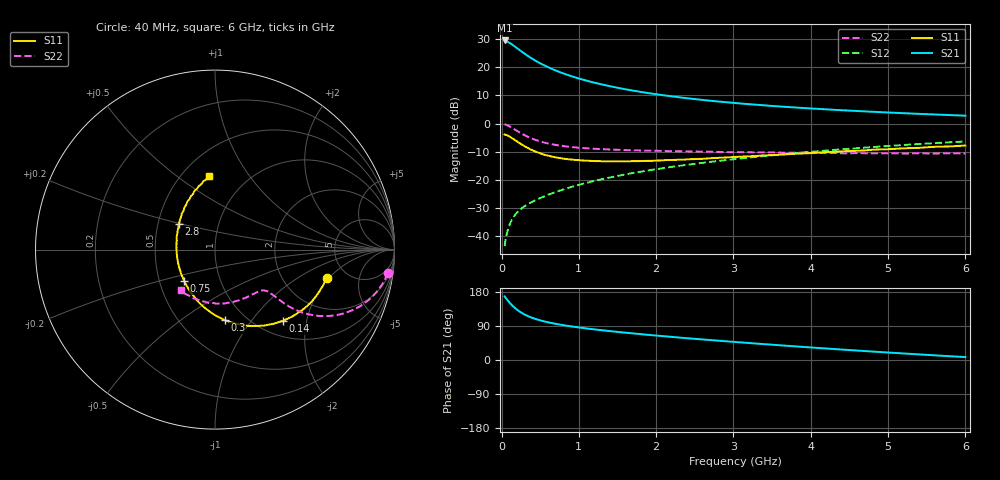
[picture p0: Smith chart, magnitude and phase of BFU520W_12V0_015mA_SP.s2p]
! Filename:  P:\Prog\Test\Noise\ATS_data\Testdata_Net\Run2\BFU520W_APM2013_06_A05_12p0V_015mA_SP_CM01_D.s2p
! Date/Time: Tue 26/Mar/2013 18:01:44
! BFU520W_APM2013_06_A05_12p0V_1to20mA_SP_CM01_Bias7_R.s2p
! MDIF S-parameter v. bias file
! BFU520W_APM2013_06_A05_12p0V_1to20mA_SP_CM01
! Date/time Thu Mar 21 16:35:01 2013
! VAR V_out= 12.0000
! VAR I_out= 14.9950
! VAR V_in= 0.7974
! VAR I_in= 0.1535
! Device data file deembeded for feedlines and parallel
! Original file: \Run2\BFU520W_APM2013_06_A05_12p0V_015mA_SP_CM01_R.s2p
! Feed-files: PR019V01_070313_Feed1.s2p, PR019V01_070313_Feed2.s2p
! Parallel-file: PR019V01_070313_Par.s2p
# MHz S MA R 50
!  Freq-MHz  S11-mag  S11-arg  S21-mag  S21-arg  S12-mag  S12-arg  S22-mag  S22-arg
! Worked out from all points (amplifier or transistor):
!   98 points, 40 MHz to 6 GHz, reference 50 ohm
!   highest |S21| = 29.4 dB at 40 MHz (marker M1)
!   |S21| within 3 dB of that: start of sweep to 214.3 MHz
!   unconditionally stable (mu >= 1): 1.331 GHz to 2.538 GHz
!   at 300 MHz: K = 0.60, MSG = 27.0 dB, |S12| = -29.3 dB
!   at 1.6 GHz: K = 1.01, MAG = 14.5 dB, |S12| = -18.0 dB
!   at 6 GHz: K = 0.88, MSG = 4.6 dB, |S12| = -6.3 dB
!   S11 on the Smith chart (normalised r, x): 40 MHz: 3.50, -1.87; 140 MHz: 1.28, -1.46; 300 MHz: 0.80, -0.75; 750 MHz: 0.67, -0.25; 2.8 GHz: 0.64, +0.20; 6 GHz: 0.68, +0.66
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40  0.6411 -14.2  29.66 167.8  0.006734 82.5  0.97 -7.7
50  0.6355 -17.8  29.56 165.0  0.008316 81.4  0.9625 -9.8
90  0.602 -31.4  27.52 154.8  0.0142 76.3  0.9125 -16.9
120  0.5699 -40.8  26.09 147.8  0.0181 73.2  0.8672 -21.4
140  0.5482 -46.5  24.95 143.6  0.02044 71.5  0.8347 -24.0
180  0.5039 -57.1  22.74 136.2  0.02466 68.7  0.7722 -28.1
220  0.4636 -66.4  20.73 129.8  0.02822 67.1  0.7149 -31.2
260  0.4267 -74.6  18.88 124.4  0.03144 66.0  0.664 -33.5
300  0.3959 -82.2  17.24 119.9  0.03444 65.4  0.6207 -35.1
340  0.3697 -88.8  15.81 116.0  0.03722 65.2  0.5834 -36.2
380  0.3463 -94.9  14.55 112.7  0.03994 65.2  0.5516 -37.0
480  0.3045 -108.0  12.09 105.9  0.04662 65.8  0.4923 -37.9
600  0.2712 -121.0  10.01 99.6  0.05454 66.8  0.4442 -38.0
750  0.2457 -134.2  8.196 93.7  0.06465 67.9  0.4079 -38.0
1050  0.2219 -154.7  6.012 84.6  0.08562 69.2  0.3689 -38.8
1500  0.2141 -177.0  4.311 74.2  0.1181 69.2  0.3432 -42.1
2050  0.2215 164.0  3.233 63.6  0.1591 67.5  0.3285 -48.4
2800  0.2472 144.6  2.461 51.1  0.2172 63.6  0.315 -60.2
3100  0.2595 138.0  2.263 46.4  0.2415 61.8  0.3123 -65.1
4100  0.3064 120.5  1.819 31.7  0.3243 54.5  0.3007 -84.9
5200  0.3646 104.5  1.528 17.2  0.4172 45.0  0.2945 -109.6
6000  0.4086 94.4  1.379 7.7  0.4823 37.4  0.2949 -129.9
